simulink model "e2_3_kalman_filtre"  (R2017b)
settings: Solver=FixedStepAuto  StartTime=0.0  StopTime=30  FixedStep=fixed_step_size  RelTol=1e-3
StopFcn:
  | if AUTOLAND
  | %1_2
  | land1 = rospublisher('/tello1/land','std_msgs/Empty');
  | msg=rosmessage(land1);
  | send(land1,msg);
  | land2 = rospublisher('/tello2/land','std_msgs/Empty');
  | msg=rosmessage(land2);
  | send(land2,msg);
  | %3_4
  | land3 = rospublisher('/tello3/land','std_msgs/Empty');
  | msg=rosmessage(land3);
  | send(land3,msg);
  | land4 = rospublisher('/tello4/land','std_msgs/Empty');
  | msg=rosmessage(land4);
  | send(land4,msg);
  | %5_6
  | land5 = rospublisher('/tello5/land','std_msgs/Empty');
  | msg=rosmessage(land5);
  | send(land5,msg);
  | land6= rospublisher('/tello6/land','std_msgs/Empty');
  | msg=rosmessage(land6);
  | send(land6,msg);
  | %7_8
  | land7 = rospublisher('/tello7/land','std_msgs/Empty');
  | msg=rosmessage(land7);
  | send(land7,msg);
  | land8 = rospublisher('/tello8/land','std_msgs/Empty');
  | msg=rosmessage(land8);
  | send(land8,msg);
  | end
  | 
  | generate_cifer_datapack
  | 
  | if TELLO_PLOT
  | tello8_plot
  | end
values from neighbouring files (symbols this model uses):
  a = XMAX    (= 0.8)    [start_tello.m]
  b = YMAX    (= 1.2)    [start_tello.m]
  battery_threshold = 15    [start_tello.m]
  bb = (ZMIN*YMAX - ZMAX*YMIN)/(YMAX - YMIN)    (= -1.05)    [start_tello.m]
  fcnCmdMag = 1    [start.m]
  fcnNumber = 4    [start.m]
  fcnSinFreq = 50.0    (= 50)    [start.m]
  high_time = 5    [start.m]
  k = (ZMAX - ZMIN)/(YMAX - YMIN)    (= 0.458333333333)    [start_tello.m]
  omega = 1.0    (= 1)    [start.m]    (also in start_tello.m = 0.3)
  PARAM_C1 = 4.0    (= 4)    [start.m]
  PARAM_C2 = 0.0187    [start.m]
  PARAM_isNoiseOn = false    [start.m]
  PARAM_T_rec = ceil(5*2*pi/PARAM_w_min)    [start.m]
  PARAM_time_end = PARAM_time_start + 20    (= 23)    [start.m]
  PARAM_time_start = 3    [start.m]
  PARAM_w_max = 12    [start.m]
  PARAM_w_min = 0.5    [start.m]
  R = 1.0    (= 1)    [start.m]    (also in start_tello.m)
  sim_end_time = 15*act_end + 4    (= 475.238898038)    [start_tello.m]
  step_period = zero1_time+high_time+zero2_time+low_time    (= 18)    [start.m]
  tb2 = tb    (= 2.7)    [start_tello.m]
  tb3 = tb*2    (= 5.4)    [start_tello.m]
  tb4 = tb*3    (= 8.1)    [start_tello.m]
  tb5 = tb*4    (= 10.8)    [start_tello.m]
  tb6 = tb*5    (= 13.5)    [start_tello.m]
  tb7 = tb*6    (= 16.2)    [start_tello.m]
  tb8 = tb*7    (= 18.9)    [start_tello.m]
  TELLO1_NUM = uint8(1)    [start_tello.m]
  TELLO2_NUM = uint8(2)    [start_tello.m]
  TELLO3_NUM = uint8(3)    [start_tello.m]
  TELLO4_NUM = uint8(4)    [start_tello.m]
  TELLO5_NUM = uint8(5)    [start_tello.m]
  TELLO6_NUM = uint8(6)    [start_tello.m]
  TELLO7_NUM = uint8(7)    [start_tello.m]
  TELLO8_NUM = uint8(8)    [start_tello.m]
  UAV_NUM = 0    [start_tello.m]
  w1 = 0.4    [start_tello.m]
  w2 = 0.2    [start_tello.m]
  z_d_for_land = -0.2    [start_tello.m]
  zero1_time = 3    [start.m]
  zero2_time = 5    [start.m]
  zero3_time = 5    [start.m]
undefined symbols (not defined in the file or in its folder): DiscIntNeverNeededParam, sigbuilder_block
libraries: simulink x45, etargetslib x24, dspnetwork x24, sharedtransform x8, aerolibanimutils x1
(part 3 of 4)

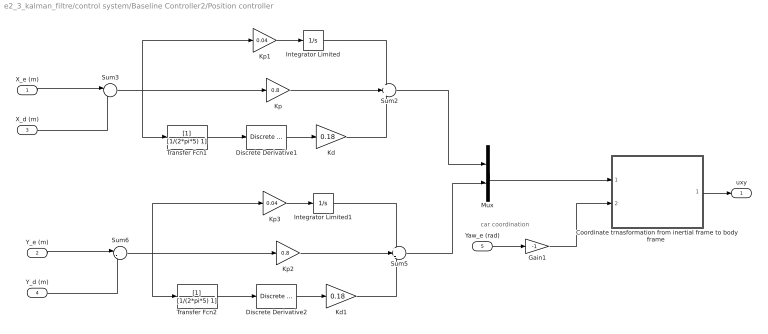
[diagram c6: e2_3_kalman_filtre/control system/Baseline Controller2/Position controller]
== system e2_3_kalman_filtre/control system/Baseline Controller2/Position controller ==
  note: car coordination
  X_e (m) : Inport
  Y_e (m) : Inport  Port=2
  X_d (m) : Inport  Port=3
  Y_d (m) : Inport  Port=4
  Yaw_e (rad) : Inport  Port=5
  "Coordinate trnasformation from inertial frame to body frame " : MATLAB Function  TreatAsAtomicUnit=on
  Discrete Derivative1 : simulink/Discrete/Discrete Derivative  gainval=1.0  ICPrevScaledInput=0.0  OutMin=[]  OutMax=[]  OutDataType=fixdt(1, 16)  OutScaling=2^-10  DoSatur=off
  Discrete Derivative2 : simulink/Discrete/Discrete Derivative  gainval=1.0  ICPrevScaledInput=0.0  OutMin=[]  OutMax=[]  OutDataType=fixdt(1, 16)  OutScaling=2^-10  DoSatur=off
  Gain1 : Gain  Gain=-1
  Integrator Limited : Integrator  LimitOutput=on  UpperSaturationLimit=0.5  LowerSaturationLimit=-0.5
  Integrator Limited1 : Integrator  LimitOutput=on  UpperSaturationLimit=0.5  LowerSaturationLimit=-0.5
  Kd : Gain  Gain=0.18
  Kd1 : Gain  Gain=0.18
  Kp : Gain  Gain=0.8
  Kp1 : Gain  Gain=0.04
  Kp2 : Gain  Gain=0.8
  Kp3 : Gain  Gain=0.04
  Mux : Mux  Inputs=2
  Sum2 : Sum  Inputs=+++
  Sum3 : Sum  Inputs=|-+
  Sum5 : Sum  Inputs=+++
  Sum6 : Sum  Inputs=|-+
  Transfer Fcn1 : TransferFcn  Denominator=[1/(2*pi*5) 1]
  Transfer Fcn2 : TransferFcn  Denominator=[1/(2*pi*5) 1]
  uxy : Outport
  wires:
  Sum6/1 -> Transfer Fcn2/1, Kp3/1, Kp2/1
  Discrete Derivative2/1 -> Kd1/1
  Kd1/1 -> Sum5/3
  Transfer Fcn2/1 -> Discrete Derivative2/1
  Y_d (m)/1 -> Sum6/2
  Transfer Fcn1/1 -> Discrete Derivative1/1
  Kd/1 -> Sum2/3
  Discrete Derivative1/1 -> Kd/1
  Sum3/1 -> Kp1/1, Transfer Fcn1/1, Kp/1
  X_d (m)/1 -> Sum3/2
  "Coordinate trnasformation from inertial frame to body frame "/1(Vec_xy) -> uxy/1
  Gain1/1 -> "Coordinate trnasformation from inertial frame to body frame "/2(psi)
  Mux/1 -> "Coordinate trnasformation from inertial frame to body frame "/1(Vec_i)
  Kp3/1 -> Integrator Limited1/1
  Sum5/1 -> Mux/2
  Integrator Limited1/1 -> Sum5/1
  Y_e (m)/1 -> Sum6/1
  Kp2/1 -> Sum5/2
  Kp/1 -> Sum2/2
  Kp1/1 -> Integrator Limited/1
  Sum2/1 -> Mux/1
  Integrator Limited/1 -> Sum2/1
  X_e (m)/1 -> Sum3/1
  Yaw_e (rad)/1 -> Gain1/1

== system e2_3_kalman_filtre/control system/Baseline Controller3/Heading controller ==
  yaw_e (rad) : Inport
  yaw_d. (rad) : Inport  Port=2
  Integrator Limited : Integrator  Commented=on  LimitOutput=on  UpperSaturationLimit=0.3  LowerSaturationLimit=-0.3
  Ki : Gain  Commented=on  Gain=0.01
  Sum1 : Sum  Inputs=|-+
  Sum2 : Sum  Inputs=|++
  proportional control gain - yaw : Gain  Gain=1.0
  yaw_rate_d. (rad/s) : Outport
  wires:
  Sum1/1 -> Ki/1, proportional control gain - yaw/1
  yaw_e (rad)/1 -> Sum1/1
  yaw_d. (rad)/1 -> Sum1/2
  proportional control gain - yaw/1 -> Sum2/1
  Integrator Limited/1 -> Sum2/2
  Ki/1 -> Integrator Limited/1
  Sum2/1 -> yaw_rate_d. (rad/s)/1

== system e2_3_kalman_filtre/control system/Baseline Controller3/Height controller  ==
  Z_d. (m) : Inport
  Z_e (m) : Inport  Port=2
  V_z : Inport  Port=3
  Integrator Limited : Integrator  LimitOutput=on  UpperSaturationLimit=0.5  LowerSaturationLimit=-0.5
  Kd : Gain  Gain=0.01
  Kp : Gain  Gain=1.0
  Kp1 : Gain  Gain=0.01
  Sum1 : Sum  Inputs=|-+
  Sum2 : Sum  Inputs=+++
  Sum3 : Sum  Inputs=|-+
  Transfer Fcn1 : TransferFcn  Denominator=[1/(2*pi*10) 1]
  Z_velocity_d (m/s) : Outport
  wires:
  Sum3/1 -> Kp1/1, Kp/1
  Z_e (m)/1 -> Sum3/1
  V_z/1 -> Transfer Fcn1/1
  Sum1/1 -> Kd/1
  Sum2/1 -> Z_velocity_d (m/s)/1
  Kp/1 -> Sum2/2
  Kd/1 -> Sum2/3
  Kp1/1 -> Integrator Limited/1
  Integrator Limited/1 -> Sum2/1
  Transfer Fcn1/1 -> Sum1/1
  Z_d. (m)/1 -> Sum3/2

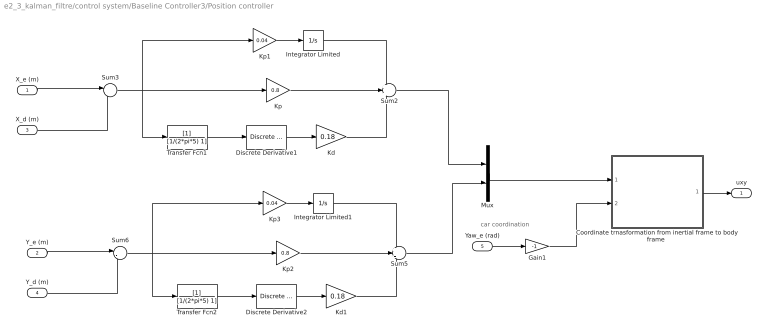
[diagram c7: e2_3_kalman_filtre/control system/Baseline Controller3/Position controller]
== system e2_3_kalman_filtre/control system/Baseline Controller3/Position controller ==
  note: car coordination
  X_e (m) : Inport
  Y_e (m) : Inport  Port=2
  X_d (m) : Inport  Port=3
  Y_d (m) : Inport  Port=4
  Yaw_e (rad) : Inport  Port=5
  "Coordinate trnasformation from inertial frame to body frame " : MATLAB Function  TreatAsAtomicUnit=on
  Discrete Derivative1 : simulink/Discrete/Discrete Derivative  gainval=1.0  ICPrevScaledInput=0.0  OutMin=[]  OutMax=[]  OutDataType=fixdt(1, 16)  OutScaling=2^-10  DoSatur=off
  Discrete Derivative2 : simulink/Discrete/Discrete Derivative  gainval=1.0  ICPrevScaledInput=0.0  OutMin=[]  OutMax=[]  OutDataType=fixdt(1, 16)  OutScaling=2^-10  DoSatur=off
  Gain1 : Gain  Gain=-1
  Integrator Limited : Integrator  LimitOutput=on  UpperSaturationLimit=0.5  LowerSaturationLimit=-0.5
  Integrator Limited1 : Integrator  LimitOutput=on  UpperSaturationLimit=0.5  LowerSaturationLimit=-0.5
  Kd : Gain  Gain=0.18
  Kd1 : Gain  Gain=0.18
  Kp : Gain  Gain=0.8
  Kp1 : Gain  Gain=0.04
  Kp2 : Gain  Gain=0.8
  Kp3 : Gain  Gain=0.04
  Mux : Mux  Inputs=2
  Sum2 : Sum  Inputs=+++
  Sum3 : Sum  Inputs=|-+
  Sum5 : Sum  Inputs=+++
  Sum6 : Sum  Inputs=|-+
  Transfer Fcn1 : TransferFcn  Denominator=[1/(2*pi*5) 1]
  Transfer Fcn2 : TransferFcn  Denominator=[1/(2*pi*5) 1]
  uxy : Outport
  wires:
  Yaw_e (rad)/1 -> Gain1/1
  X_e (m)/1 -> Sum3/1
  Integrator Limited/1 -> Sum2/1
  Sum2/1 -> Mux/1
  Kp1/1 -> Integrator Limited/1
  Kp/1 -> Sum2/2
  Kp2/1 -> Sum5/2
  Y_e (m)/1 -> Sum6/1
  Integrator Limited1/1 -> Sum5/1
  Sum5/1 -> Mux/2
  Kp3/1 -> Integrator Limited1/1
  Mux/1 -> "Coordinate trnasformation from inertial frame to body frame "/1(Vec_i)
  Gain1/1 -> "Coordinate trnasformation from inertial frame to body frame "/2(psi)
  "Coordinate trnasformation from inertial frame to body frame "/1(Vec_xy) -> uxy/1
  X_d (m)/1 -> Sum3/2
  Sum3/1 -> Kp/1, Transfer Fcn1/1, Kp1/1
  Discrete Derivative1/1 -> Kd/1
  Kd/1 -> Sum2/3
  Transfer Fcn1/1 -> Discrete Derivative1/1
  Y_d (m)/1 -> Sum6/2
  Transfer Fcn2/1 -> Discrete Derivative2/1
  Kd1/1 -> Sum5/3
  Discrete Derivative2/1 -> Kd1/1
  Sum6/1 -> Kp2/1, Kp3/1, Transfer Fcn2/1

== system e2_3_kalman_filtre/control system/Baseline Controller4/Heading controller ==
  yaw_e (rad) : Inport
  yaw_d. (rad) : Inport  Port=2
  Integrator Limited : Integrator  Commented=on  LimitOutput=on  UpperSaturationLimit=0.3  LowerSaturationLimit=-0.3
  Ki : Gain  Commented=on  Gain=0.01
  Sum1 : Sum  Inputs=|-+
  Sum2 : Sum  Inputs=|++
  proportional control gain - yaw : Gain  Gain=1.0
  yaw_rate_d. (rad/s) : Outport
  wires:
  Sum2/1 -> yaw_rate_d. (rad/s)/1
  Ki/1 -> Integrator Limited/1
  Integrator Limited/1 -> Sum2/2
  proportional control gain - yaw/1 -> Sum2/1
  yaw_d. (rad)/1 -> Sum1/2
  yaw_e (rad)/1 -> Sum1/1
  Sum1/1 -> proportional control gain - yaw/1, Ki/1

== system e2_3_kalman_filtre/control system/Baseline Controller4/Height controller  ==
  Z_d. (m) : Inport
  Z_e (m) : Inport  Port=2
  V_z : Inport  Port=3
  Integrator Limited : Integrator  LimitOutput=on  UpperSaturationLimit=0.5  LowerSaturationLimit=-0.5
  Kd : Gain  Gain=0.01
  Kp : Gain  Gain=1.0
  Kp1 : Gain  Gain=0.01
  Sum1 : Sum  Inputs=|-+
  Sum2 : Sum  Inputs=+++
  Sum3 : Sum  Inputs=|-+
  Transfer Fcn1 : TransferFcn  Denominator=[1/(2*pi*10) 1]
  Z_velocity_d (m/s) : Outport
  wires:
  Z_d. (m)/1 -> Sum3/2
  Transfer Fcn1/1 -> Sum1/1
  Integrator Limited/1 -> Sum2/1
  Kp1/1 -> Integrator Limited/1
  Kd/1 -> Sum2/3
  Kp/1 -> Sum2/2
  Sum2/1 -> Z_velocity_d (m/s)/1
  Sum1/1 -> Kd/1
  V_z/1 -> Transfer Fcn1/1
  Z_e (m)/1 -> Sum3/1
  Sum3/1 -> Kp/1, Kp1/1

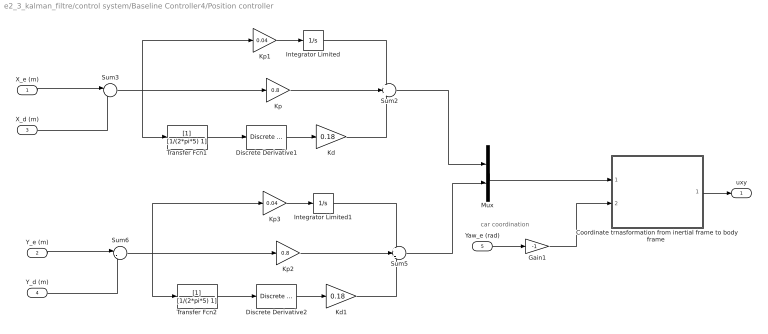
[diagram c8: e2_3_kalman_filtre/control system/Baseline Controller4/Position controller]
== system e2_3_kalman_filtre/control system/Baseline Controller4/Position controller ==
  note: car coordination
  X_e (m) : Inport
  Y_e (m) : Inport  Port=2
  X_d (m) : Inport  Port=3
  Y_d (m) : Inport  Port=4
  Yaw_e (rad) : Inport  Port=5
  "Coordinate trnasformation from inertial frame to body frame " : MATLAB Function  TreatAsAtomicUnit=on
  Discrete Derivative1 : simulink/Discrete/Discrete Derivative  gainval=1.0  ICPrevScaledInput=0.0  OutMin=[]  OutMax=[]  OutDataType=fixdt(1, 16)  OutScaling=2^-10  DoSatur=off
  Discrete Derivative2 : simulink/Discrete/Discrete Derivative  gainval=1.0  ICPrevScaledInput=0.0  OutMin=[]  OutMax=[]  OutDataType=fixdt(1, 16)  OutScaling=2^-10  DoSatur=off
  Gain1 : Gain  Gain=-1
  Integrator Limited : Integrator  LimitOutput=on  UpperSaturationLimit=0.5  LowerSaturationLimit=-0.5
  Integrator Limited1 : Integrator  LimitOutput=on  UpperSaturationLimit=0.5  LowerSaturationLimit=-0.5
  Kd : Gain  Gain=0.18
  Kd1 : Gain  Gain=0.18
  Kp : Gain  Gain=0.8
  Kp1 : Gain  Gain=0.04
  Kp2 : Gain  Gain=0.8
  Kp3 : Gain  Gain=0.04
  Mux : Mux  Inputs=2
  Sum2 : Sum  Inputs=+++
  Sum3 : Sum  Inputs=|-+
  Sum5 : Sum  Inputs=+++
  Sum6 : Sum  Inputs=|-+
  Transfer Fcn1 : TransferFcn  Denominator=[1/(2*pi*5) 1]
  Transfer Fcn2 : TransferFcn  Denominator=[1/(2*pi*5) 1]
  uxy : Outport
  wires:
  Sum6/1 -> Transfer Fcn2/1, Kp3/1, Kp2/1
  Discrete Derivative2/1 -> Kd1/1
  Kd1/1 -> Sum5/3
  Transfer Fcn2/1 -> Discrete Derivative2/1
  Y_d (m)/1 -> Sum6/2
  Transfer Fcn1/1 -> Discrete Derivative1/1
  Kd/1 -> Sum2/3
  Discrete Derivative1/1 -> Kd/1
  Sum3/1 -> Kp1/1, Transfer Fcn1/1, Kp/1
  X_d (m)/1 -> Sum3/2
  "Coordinate trnasformation from inertial frame to body frame "/1(Vec_xy) -> uxy/1
  Gain1/1 -> "Coordinate trnasformation from inertial frame to body frame "/2(psi)
  Mux/1 -> "Coordinate trnasformation from inertial frame to body frame "/1(Vec_i)
  Kp3/1 -> Integrator Limited1/1
  Sum5/1 -> Mux/2
  Integrator Limited1/1 -> Sum5/1
  Y_e (m)/1 -> Sum6/1
  Kp2/1 -> Sum5/2
  Kp/1 -> Sum2/2
  Kp1/1 -> Integrator Limited/1
  Sum2/1 -> Mux/1
  Integrator Limited/1 -> Sum2/1
  X_e (m)/1 -> Sum3/1
  Yaw_e (rad)/1 -> Gain1/1

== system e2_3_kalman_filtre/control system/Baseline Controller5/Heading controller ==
  yaw_e (rad) : Inport
  yaw_d. (rad) : Inport  Port=2
  Integrator Limited : Integrator  Commented=on  LimitOutput=on  UpperSaturationLimit=0.3  LowerSaturationLimit=-0.3
  Ki : Gain  Commented=on  Gain=0.01
  Sum1 : Sum  Inputs=|-+
  Sum2 : Sum  Inputs=|++
  proportional control gain - yaw : Gain  Gain=1.0
  yaw_rate_d. (rad/s) : Outport
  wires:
  Sum1/1 -> Ki/1, proportional control gain - yaw/1
  yaw_e (rad)/1 -> Sum1/1
  yaw_d. (rad)/1 -> Sum1/2
  proportional control gain - yaw/1 -> Sum2/1
  Integrator Limited/1 -> Sum2/2
  Ki/1 -> Integrator Limited/1
  Sum2/1 -> yaw_rate_d. (rad/s)/1

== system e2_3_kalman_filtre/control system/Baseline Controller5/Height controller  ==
  Z_d. (m) : Inport
  Z_e (m) : Inport  Port=2
  V_z : Inport  Port=3
  Integrator Limited : Integrator  LimitOutput=on  UpperSaturationLimit=0.5  LowerSaturationLimit=-0.5
  Kd : Gain  Gain=0.01
  Kp : Gain  Gain=1.0
  Kp1 : Gain  Gain=0.01
  Sum1 : Sum  Inputs=|-+
  Sum2 : Sum  Inputs=+++
  Sum3 : Sum  Inputs=|-+
  Transfer Fcn1 : TransferFcn  Denominator=[1/(2*pi*10) 1]
  Z_velocity_d (m/s) : Outport
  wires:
  Sum3/1 -> Kp1/1, Kp/1
  Z_e (m)/1 -> Sum3/1
  V_z/1 -> Transfer Fcn1/1
  Sum1/1 -> Kd/1
  Sum2/1 -> Z_velocity_d (m/s)/1
  Kp/1 -> Sum2/2
  Kd/1 -> Sum2/3
  Kp1/1 -> Integrator Limited/1
  Integrator Limited/1 -> Sum2/1
  Transfer Fcn1/1 -> Sum1/1
  Z_d. (m)/1 -> Sum3/2

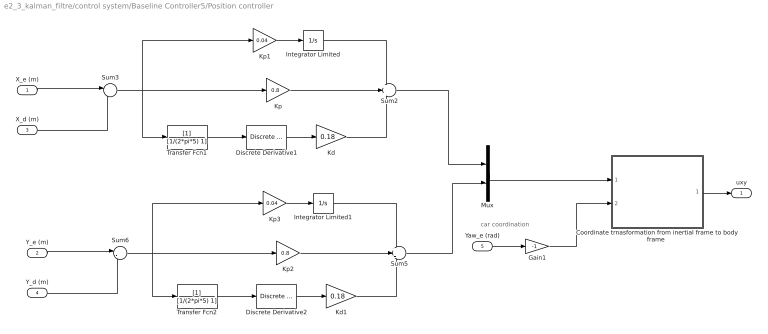
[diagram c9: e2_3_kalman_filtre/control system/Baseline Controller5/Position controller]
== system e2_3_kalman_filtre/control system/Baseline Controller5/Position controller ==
  note: car coordination
  X_e (m) : Inport
  Y_e (m) : Inport  Port=2
  X_d (m) : Inport  Port=3
  Y_d (m) : Inport  Port=4
  Yaw_e (rad) : Inport  Port=5
  "Coordinate trnasformation from inertial frame to body frame " : MATLAB Function  TreatAsAtomicUnit=on
  Discrete Derivative1 : simulink/Discrete/Discrete Derivative  gainval=1.0  ICPrevScaledInput=0.0  OutMin=[]  OutMax=[]  OutDataType=fixdt(1, 16)  OutScaling=2^-10  DoSatur=off
  Discrete Derivative2 : simulink/Discrete/Discrete Derivative  gainval=1.0  ICPrevScaledInput=0.0  OutMin=[]  OutMax=[]  OutDataType=fixdt(1, 16)  OutScaling=2^-10  DoSatur=off
  Gain1 : Gain  Gain=-1
  Integrator Limited : Integrator  LimitOutput=on  UpperSaturationLimit=0.5  LowerSaturationLimit=-0.5
  Integrator Limited1 : Integrator  LimitOutput=on  UpperSaturationLimit=0.5  LowerSaturationLimit=-0.5
  Kd : Gain  Gain=0.18
  Kd1 : Gain  Gain=0.18
  Kp : Gain  Gain=0.8
  Kp1 : Gain  Gain=0.04
  Kp2 : Gain  Gain=0.8
  Kp3 : Gain  Gain=0.04
  Mux : Mux  Inputs=2
  Sum2 : Sum  Inputs=+++
  Sum3 : Sum  Inputs=|-+
  Sum5 : Sum  Inputs=+++
  Sum6 : Sum  Inputs=|-+
  Transfer Fcn1 : TransferFcn  Denominator=[1/(2*pi*5) 1]
  Transfer Fcn2 : TransferFcn  Denominator=[1/(2*pi*5) 1]
  uxy : Outport
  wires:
  Yaw_e (rad)/1 -> Gain1/1
  X_e (m)/1 -> Sum3/1
  Integrator Limited/1 -> Sum2/1
  Sum2/1 -> Mux/1
  Kp1/1 -> Integrator Limited/1
  Kp/1 -> Sum2/2
  Kp2/1 -> Sum5/2
  Y_e (m)/1 -> Sum6/1
  Integrator Limited1/1 -> Sum5/1
  Sum5/1 -> Mux/2
  Kp3/1 -> Integrator Limited1/1
  Mux/1 -> "Coordinate trnasformation from inertial frame to body frame "/1(Vec_i)
  Gain1/1 -> "Coordinate trnasformation from inertial frame to body frame "/2(psi)
  "Coordinate trnasformation from inertial frame to body frame "/1(Vec_xy) -> uxy/1
  X_d (m)/1 -> Sum3/2
  Sum3/1 -> Kp/1, Transfer Fcn1/1, Kp1/1
  Discrete Derivative1/1 -> Kd/1
  Kd/1 -> Sum2/3
  Transfer Fcn1/1 -> Discrete Derivative1/1
  Y_d (m)/1 -> Sum6/2
  Transfer Fcn2/1 -> Discrete Derivative2/1
  Kd1/1 -> Sum5/3
  Discrete Derivative2/1 -> Kd1/1
  Sum6/1 -> Kp2/1, Kp3/1, Transfer Fcn2/1

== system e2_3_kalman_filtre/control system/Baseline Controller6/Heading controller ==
  yaw_e (rad) : Inport
  yaw_d. (rad) : Inport  Port=2
  Integrator Limited : Integrator  Commented=on  LimitOutput=on  UpperSaturationLimit=0.3  LowerSaturationLimit=-0.3
  Ki : Gain  Commented=on  Gain=0.01
  Sum1 : Sum  Inputs=|-+
  Sum2 : Sum  Inputs=|++
  proportional control gain - yaw : Gain  Gain=1.0
  yaw_rate_d. (rad/s) : Outport
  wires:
  Sum2/1 -> yaw_rate_d. (rad/s)/1
  Ki/1 -> Integrator Limited/1
  Integrator Limited/1 -> Sum2/2
  proportional control gain - yaw/1 -> Sum2/1
  yaw_d. (rad)/1 -> Sum1/2
  yaw_e (rad)/1 -> Sum1/1
  Sum1/1 -> proportional control gain - yaw/1, Ki/1

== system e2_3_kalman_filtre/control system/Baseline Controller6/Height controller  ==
  Z_d. (m) : Inport
  Z_e (m) : Inport  Port=2
  V_z : Inport  Port=3
  Integrator Limited : Integrator  LimitOutput=on  UpperSaturationLimit=0.5  LowerSaturationLimit=-0.5
  Kd : Gain  Gain=0.01
  Kp : Gain  Gain=1.0
  Kp1 : Gain  Gain=0.01
  Sum1 : Sum  Inputs=|-+
  Sum2 : Sum  Inputs=+++
  Sum3 : Sum  Inputs=|-+
  Transfer Fcn1 : TransferFcn  Denominator=[1/(2*pi*10) 1]
  Z_velocity_d (m/s) : Outport
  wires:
  Z_d. (m)/1 -> Sum3/2
  Transfer Fcn1/1 -> Sum1/1
  Integrator Limited/1 -> Sum2/1
  Kp1/1 -> Integrator Limited/1
  Kd/1 -> Sum2/3
  Kp/1 -> Sum2/2
  Sum2/1 -> Z_velocity_d (m/s)/1
  Sum1/1 -> Kd/1
  V_z/1 -> Transfer Fcn1/1
  Z_e (m)/1 -> Sum3/1
  Sum3/1 -> Kp/1, Kp1/1

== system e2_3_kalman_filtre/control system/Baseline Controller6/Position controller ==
  note: car coordination
  X_e (m) : Inport
  Y_e (m) : Inport  Port=2
  X_d (m) : Inport  Port=3
  Y_d (m) : Inport  Port=4
  Yaw_e (rad) : Inport  Port=5
  "Coordinate trnasformation from inertial frame to body frame " : MATLAB Function  TreatAsAtomicUnit=on
  Discrete Derivative1 : simulink/Discrete/Discrete Derivative  gainval=1.0  ICPrevScaledInput=0.0  OutMin=[]  OutMax=[]  OutDataType=fixdt(1, 16)  OutScaling=2^-10  DoSatur=off
  Discrete Derivative2 : simulink/Discrete/Discrete Derivative  gainval=1.0  ICPrevScaledInput=0.0  OutMin=[]  OutMax=[]  OutDataType=fixdt(1, 16)  OutScaling=2^-10  DoSatur=off
  Gain1 : Gain  Gain=-1
  Integrator Limited : Integrator  LimitOutput=on  UpperSaturationLimit=0.5  LowerSaturationLimit=-0.5
  Integrator Limited1 : Integrator  LimitOutput=on  UpperSaturationLimit=0.5  LowerSaturationLimit=-0.5
  Kd : Gain  Gain=0.18
  Kd1 : Gain  Gain=0.18
  Kp : Gain  Gain=0.8
  Kp1 : Gain  Gain=0.04
  Kp2 : Gain  Gain=0.8
  Kp3 : Gain  Gain=0.04
  Mux : Mux  Inputs=2
  Sum2 : Sum  Inputs=+++
  Sum3 : Sum  Inputs=|-+
  Sum5 : Sum  Inputs=+++
  Sum6 : Sum  Inputs=|-+
  Transfer Fcn1 : TransferFcn  Denominator=[1/(2*pi*5) 1]
  Transfer Fcn2 : TransferFcn  Denominator=[1/(2*pi*5) 1]
  uxy : Outport
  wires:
  Sum6/1 -> Transfer Fcn2/1, Kp3/1, Kp2/1
  Discrete Derivative2/1 -> Kd1/1
  Kd1/1 -> Sum5/3
  Transfer Fcn2/1 -> Discrete Derivative2/1
  Y_d (m)/1 -> Sum6/2
  Transfer Fcn1/1 -> Discrete Derivative1/1
  Kd/1 -> Sum2/3
  Discrete Derivative1/1 -> Kd/1
  Sum3/1 -> Kp1/1, Transfer Fcn1/1, Kp/1
  X_d (m)/1 -> Sum3/2
  "Coordinate trnasformation from inertial frame to body frame "/1(Vec_xy) -> uxy/1
  Gain1/1 -> "Coordinate trnasformation from inertial frame to body frame "/2(psi)
  Mux/1 -> "Coordinate trnasformation from inertial frame to body frame "/1(Vec_i)
  Kp3/1 -> Integrator Limited1/1
  Sum5/1 -> Mux/2
  Integrator Limited1/1 -> Sum5/1
  Y_e (m)/1 -> Sum6/1
  Kp2/1 -> Sum5/2
  Kp/1 -> Sum2/2
  Kp1/1 -> Integrator Limited/1
  Sum2/1 -> Mux/1
  Integrator Limited/1 -> Sum2/1
  X_e (m)/1 -> Sum3/1
  Yaw_e (rad)/1 -> Gain1/1

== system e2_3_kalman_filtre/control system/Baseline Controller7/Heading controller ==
  yaw_e (rad) : Inport
  yaw_d. (rad) : Inport  Port=2
  Integrator Limited : Integrator  Commented=on  LimitOutput=on  UpperSaturationLimit=0.3  LowerSaturationLimit=-0.3
  Ki : Gain  Commented=on  Gain=0.01
  Sum1 : Sum  Inputs=|-+
  Sum2 : Sum  Inputs=|++
  proportional control gain - yaw : Gain  Gain=1.0
  yaw_rate_d. (rad/s) : Outport
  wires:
  Sum1/1 -> Ki/1, proportional control gain - yaw/1
  yaw_e (rad)/1 -> Sum1/1
  yaw_d. (rad)/1 -> Sum1/2
  proportional control gain - yaw/1 -> Sum2/1
  Integrator Limited/1 -> Sum2/2
  Ki/1 -> Integrator Limited/1
  Sum2/1 -> yaw_rate_d. (rad/s)/1

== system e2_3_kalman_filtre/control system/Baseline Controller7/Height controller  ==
  Z_d. (m) : Inport
  Z_e (m) : Inport  Port=2
  V_z : Inport  Port=3
  Integrator Limited : Integrator  LimitOutput=on  UpperSaturationLimit=0.5  LowerSaturationLimit=-0.5
  Kd : Gain  Gain=0.01
  Kp : Gain  Gain=1.0
  Kp1 : Gain  Gain=0.01
  Sum1 : Sum  Inputs=|-+
  Sum2 : Sum  Inputs=+++
  Sum3 : Sum  Inputs=|-+
  Transfer Fcn1 : TransferFcn  Denominator=[1/(2*pi*10) 1]
  Z_velocity_d (m/s) : Outport
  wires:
  Sum3/1 -> Kp1/1, Kp/1
  Z_e (m)/1 -> Sum3/1
  V_z/1 -> Transfer Fcn1/1
  Sum1/1 -> Kd/1
  Sum2/1 -> Z_velocity_d (m/s)/1
  Kp/1 -> Sum2/2
  Kd/1 -> Sum2/3
  Kp1/1 -> Integrator Limited/1
  Integrator Limited/1 -> Sum2/1
  Transfer Fcn1/1 -> Sum1/1
  Z_d. (m)/1 -> Sum3/2

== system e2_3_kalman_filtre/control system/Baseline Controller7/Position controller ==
  note: car coordination
  X_e (m) : Inport
  Y_e (m) : Inport  Port=2
  X_d (m) : Inport  Port=3
  Y_d (m) : Inport  Port=4
  Yaw_e (rad) : Inport  Port=5
  "Coordinate trnasformation from inertial frame to body frame " : MATLAB Function  TreatAsAtomicUnit=on
  Discrete Derivative1 : simulink/Discrete/Discrete Derivative  gainval=1.0  ICPrevScaledInput=0.0  OutMin=[]  OutMax=[]  OutDataType=fixdt(1, 16)  OutScaling=2^-10  DoSatur=off
  Discrete Derivative2 : simulink/Discrete/Discrete Derivative  gainval=1.0  ICPrevScaledInput=0.0  OutMin=[]  OutMax=[]  OutDataType=fixdt(1, 16)  OutScaling=2^-10  DoSatur=off
  Gain1 : Gain  Gain=-1
  Integrator Limited : Integrator  LimitOutput=on  UpperSaturationLimit=0.5  LowerSaturationLimit=-0.5
  Integrator Limited1 : Integrator  LimitOutput=on  UpperSaturationLimit=0.5  LowerSaturationLimit=-0.5
  Kd : Gain  Gain=0.18
  Kd1 : Gain  Gain=0.18
  Kp : Gain  Gain=0.8
  Kp1 : Gain  Gain=0.04
  Kp2 : Gain  Gain=0.8
  Kp3 : Gain  Gain=0.04
  Mux : Mux  Inputs=2
  Sum2 : Sum  Inputs=+++
  Sum3 : Sum  Inputs=|-+
  Sum5 : Sum  Inputs=+++
  Sum6 : Sum  Inputs=|-+
  Transfer Fcn1 : TransferFcn  Denominator=[1/(2*pi*5) 1]
  Transfer Fcn2 : TransferFcn  Denominator=[1/(2*pi*5) 1]
  uxy : Outport
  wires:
  Yaw_e (rad)/1 -> Gain1/1
  X_e (m)/1 -> Sum3/1
  Integrator Limited/1 -> Sum2/1
  Sum2/1 -> Mux/1
  Kp1/1 -> Integrator Limited/1
  Kp/1 -> Sum2/2
  Kp2/1 -> Sum5/2
  Y_e (m)/1 -> Sum6/1
  Integrator Limited1/1 -> Sum5/1
  Sum5/1 -> Mux/2
  Kp3/1 -> Integrator Limited1/1
  Mux/1 -> "Coordinate trnasformation from inertial frame to body frame "/1(Vec_i)
  Gain1/1 -> "Coordinate trnasformation from inertial frame to body frame "/2(psi)
  "Coordinate trnasformation from inertial frame to body frame "/1(Vec_xy) -> uxy/1
  X_d (m)/1 -> Sum3/2
  Sum3/1 -> Kp/1, Transfer Fcn1/1, Kp1/1
  Discrete Derivative1/1 -> Kd/1
  Kd/1 -> Sum2/3
  Transfer Fcn1/1 -> Discrete Derivative1/1
  Y_d (m)/1 -> Sum6/2
  Transfer Fcn2/1 -> Discrete Derivative2/1
  Kd1/1 -> Sum5/3
  Discrete Derivative2/1 -> Kd1/1
  Sum6/1 -> Kp2/1, Kp3/1, Transfer Fcn2/1

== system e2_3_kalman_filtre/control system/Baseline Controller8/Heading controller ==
  yaw_e (rad) : Inport
  yaw_d. (rad) : Inport  Port=2
  Integrator Limited : Integrator  Commented=on  LimitOutput=on  UpperSaturationLimit=0.3  LowerSaturationLimit=-0.3
  Ki : Gain  Commented=on  Gain=0.01
  Sum1 : Sum  Inputs=|-+
  Sum2 : Sum  Inputs=|++
  proportional control gain - yaw : Gain  Gain=1.0
  yaw_rate_d. (rad/s) : Outport
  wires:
  Sum2/1 -> yaw_rate_d. (rad/s)/1
  Ki/1 -> Integrator Limited/1
  Integrator Limited/1 -> Sum2/2
  proportional control gain - yaw/1 -> Sum2/1
  yaw_d. (rad)/1 -> Sum1/2
  yaw_e (rad)/1 -> Sum1/1
  Sum1/1 -> proportional control gain - yaw/1, Ki/1

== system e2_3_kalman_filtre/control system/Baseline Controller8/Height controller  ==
  Z_d. (m) : Inport
  Z_e (m) : Inport  Port=2
  V_z : Inport  Port=3
  Integrator Limited : Integrator  LimitOutput=on  UpperSaturationLimit=0.5  LowerSaturationLimit=-0.5
  Kd : Gain  Gain=0.01
  Kp : Gain  Gain=1.0
  Kp1 : Gain  Gain=0.01
  Sum1 : Sum  Inputs=|-+
  Sum2 : Sum  Inputs=+++
  Sum3 : Sum  Inputs=|-+
  Transfer Fcn1 : TransferFcn  Denominator=[1/(2*pi*10) 1]
  Z_velocity_d (m/s) : Outport
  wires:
  Z_d. (m)/1 -> Sum3/2
  Transfer Fcn1/1 -> Sum1/1
  Integrator Limited/1 -> Sum2/1
  Kp1/1 -> Integrator Limited/1
  Kd/1 -> Sum2/3
  Kp/1 -> Sum2/2
  Sum2/1 -> Z_velocity_d (m/s)/1
  Sum1/1 -> Kd/1
  V_z/1 -> Transfer Fcn1/1
  Z_e (m)/1 -> Sum3/1
  Sum3/1 -> Kp/1, Kp1/1

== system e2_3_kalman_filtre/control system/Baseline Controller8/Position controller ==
  note: car coordination
  X_e (m) : Inport
  Y_e (m) : Inport  Port=2
  X_d (m) : Inport  Port=3
  Y_d (m) : Inport  Port=4
  Yaw_e (rad) : Inport  Port=5
  "Coordinate trnasformation from inertial frame to body frame " : MATLAB Function  TreatAsAtomicUnit=on
  Discrete Derivative1 : simulink/Discrete/Discrete Derivative  gainval=1.0  ICPrevScaledInput=0.0  OutMin=[]  OutMax=[]  OutDataType=fixdt(1, 16)  OutScaling=2^-10  DoSatur=off
  Discrete Derivative2 : simulink/Discrete/Discrete Derivative  gainval=1.0  ICPrevScaledInput=0.0  OutMin=[]  OutMax=[]  OutDataType=fixdt(1, 16)  OutScaling=2^-10  DoSatur=off
  Gain1 : Gain  Gain=-1
  Integrator Limited : Integrator  LimitOutput=on  UpperSaturationLimit=0.5  LowerSaturationLimit=-0.5
  Integrator Limited1 : Integrator  LimitOutput=on  UpperSaturationLimit=0.5  LowerSaturationLimit=-0.5
  Kd : Gain  Gain=0.18
  Kd1 : Gain  Gain=0.18
  Kp : Gain  Gain=0.8
  Kp1 : Gain  Gain=0.04
  Kp2 : Gain  Gain=0.8
  Kp3 : Gain  Gain=0.04
  Mux : Mux  Inputs=2
  Sum2 : Sum  Inputs=+++
  Sum3 : Sum  Inputs=|-+
  Sum5 : Sum  Inputs=+++
  Sum6 : Sum  Inputs=|-+
  Transfer Fcn1 : TransferFcn  Denominator=[1/(2*pi*5) 1]
  Transfer Fcn2 : TransferFcn  Denominator=[1/(2*pi*5) 1]
  uxy : Outport
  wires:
  Sum6/1 -> Transfer Fcn2/1, Kp3/1, Kp2/1
  Discrete Derivative2/1 -> Kd1/1
  Kd1/1 -> Sum5/3
  Transfer Fcn2/1 -> Discrete Derivative2/1
  Y_d (m)/1 -> Sum6/2
  Transfer Fcn1/1 -> Discrete Derivative1/1
  Kd/1 -> Sum2/3
  Discrete Derivative1/1 -> Kd/1
  Sum3/1 -> Kp1/1, Transfer Fcn1/1, Kp/1
  X_d (m)/1 -> Sum3/2
  "Coordinate trnasformation from inertial frame to body frame "/1(Vec_xy) -> uxy/1
  Gain1/1 -> "Coordinate trnasformation from inertial frame to body frame "/2(psi)
  Mux/1 -> "Coordinate trnasformation from inertial frame to body frame "/1(Vec_i)
  Kp3/1 -> Integrator Limited1/1
  Sum5/1 -> Mux/2
  Integrator Limited1/1 -> Sum5/1
  Y_e (m)/1 -> Sum6/1
  Kp2/1 -> Sum5/2
  Kp/1 -> Sum2/2
  Kp1/1 -> Integrator Limited/1
  Sum2/1 -> Mux/1
  Integrator Limited/1 -> Sum2/1
  X_e (m)/1 -> Sum3/1
  Yaw_e (rad)/1 -> Gain1/1

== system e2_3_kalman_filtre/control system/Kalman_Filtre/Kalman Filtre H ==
  The system output: Position : Inport
  real_vz : Inport  Port=2
  Demux : Demux  Outputs=9
  Error : Scope
  Kalman Filtre H : Subsystem
  Kalman Filtre for getting the velocity H : MATLAB Function  TreatAsAtomicUnit=on
  Manual Switch1 : ManualSwitch  CurrentSetting=0
  Memory block for resolving the 'algebraic loop' problem : Memory
  Scope2 : Scope
  Scope4 : Scope  NumInputPorts=8
  Sum : Sum  Inputs=-+|
  The comparison of velocity signal between 'Derivative' and 'Kalman filtering' : Scope  NumInputPorts=2
  Unit Delay1 : UnitDelay  SampleTime=-1
  Unit Delay7 : UnitDelay  SampleTime=-1
  Unit Delay8 : UnitDelay  SampleTime=-1
  Zero-Order Hold1 : ZeroOrderHold  SampleTime=-1
  Out velocity feedback : Outport
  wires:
  Kalman Filtre for getting the velocity H/1(Covariance_matrice) -> Scope2/1
  Kalman Filtre for getting the velocity H/2(X_Kalmanfiltred) -> Memory block for resolving the 'algebraic loop' problem/1
  Memory block for resolving the 'algebraic loop' problem/1 -> Demux/1
  Zero-Order Hold1/1 -> Kalman Filtre for getting the velocity H/1(Mesurement_Velocity)
  Manual Switch1/1 -> Out velocity feedback/1
  Demux/1 -> Scope4/1
  The system output: Position/1 -> Kalman Filtre H/1(The system output: Position), Unit Delay7/1
  Demux/2 -> Scope4/2
  Demux/3 -> Scope4/3
  Demux/4 -> Scope4/4
  Demux/5 -> Scope4/5
  Unit Delay8/1 -> Zero-Order Hold1/1
  Demux/6 -> Scope4/6
  Demux/7 -> Scope4/8
  Demux/8 -> Manual Switch1/1, Sum/1, The comparison of velocity signal between 'Derivative' and 'Kalman filtering'/1
  Demux/9 -> Scope4/7
  real_vz/1 -> Manual Switch1/2, The comparison of velocity signal between 'Derivative' and 'Kalman filtering'/2
  Unit Delay7/1 -> Unit Delay1/1
  Unit Delay1/1 -> Unit Delay8/1
  Sum/1 -> Error/1
  Kalman Filtre H/1(Out velocity feedback) -> Sum/2

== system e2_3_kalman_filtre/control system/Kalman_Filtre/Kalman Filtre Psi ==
  The system output: Position : Inport
  real_vpsi : Inport  Port=2
  Demux : Demux  Outputs=9
  Error : Scope
  Kalman Filtre Psi : Subsystem
  Kalman Filtre for getting the velocity Psi : MATLAB Function  TreatAsAtomicUnit=on
  Manual Switch1 : ManualSwitch  CurrentSetting=0
  Memory block for resolving the 'algebraic loop' problem : Memory
  Scope2 : Scope
  Scope4 : Scope  NumInputPorts=8
  Sum : Sum  Inputs=-+|
  The comparison of velocity signal between 'Derivative' and 'Kalman filtering' : Scope  NumInputPorts=2
  Unit Delay1 : UnitDelay  SampleTime=-1
  Unit Delay7 : UnitDelay  SampleTime=-1
  Unit Delay8 : UnitDelay  SampleTime=-1
  Zero-Order Hold1 : ZeroOrderHold  SampleTime=-1
  Out velocity feedback : Outport
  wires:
  Kalman Filtre for getting the velocity Psi/1(Covariance_matrice) -> Scope2/1
  Kalman Filtre for getting the velocity Psi/2(X_Kalmanfiltred) -> Memory block for resolving the 'algebraic loop' problem/1
  Memory block for resolving the 'algebraic loop' problem/1 -> Demux/1
  Zero-Order Hold1/1 -> Kalman Filtre for getting the velocity Psi/1(Mesurement_Velocity)
  Manual Switch1/1 -> Out velocity feedback/1
  Demux/1 -> Scope4/1
  The system output: Position/1 -> Kalman Filtre Psi/1(The system output: Position), Unit Delay7/1
  Demux/2 -> Scope4/2
  Demux/3 -> Scope4/3
  Demux/4 -> Scope4/4
  Demux/5 -> Scope4/5
  Unit Delay8/1 -> Zero-Order Hold1/1
  Demux/6 -> Scope4/6
  Demux/7 -> Scope4/8
  Demux/8 -> Manual Switch1/1, Sum/1, The comparison of velocity signal between 'Derivative' and 'Kalman filtering'/1
  Demux/9 -> Scope4/7
  real_vpsi/1 -> Manual Switch1/2, The comparison of velocity signal between 'Derivative' and 'Kalman filtering'/2
  Unit Delay7/1 -> Unit Delay1/1
  Unit Delay1/1 -> Unit Delay8/1
  Sum/1 -> Error/1
  Kalman Filtre Psi/1(Out velocity feedback) -> Sum/2

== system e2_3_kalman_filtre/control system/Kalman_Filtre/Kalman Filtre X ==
  The system output: Position : Inport
  real_vx : Inport  Port=2
  Demux : Demux  Outputs=9
  Error : Scope
  Kalman Filtre X : Subsystem
  Kalman Filtre for getting the velocity X : MATLAB Function  TreatAsAtomicUnit=on
  Manual Switch1 : ManualSwitch  CurrentSetting=0
  Memory block for resolving the 'algebraic loop' problem : Memory
  Scope : Scope
  Scope4 : Scope  NumInputPorts=8
  Sum : Sum  Inputs=-+|
  The comparison of velocity signal between 'Derivative' and 'Kalman filtering' : Scope  NumInputPorts=3
  Unit Delay{1..2,7..8} (4 alike) : UnitDelay  SampleTime=-1
  Zero-Order Hold1 : ZeroOrderHold  SampleTime=-1
  Out velocity feedback : Outport
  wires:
  Kalman Filtre for getting the velocity X/1(Covariance_matrice) -> Scope/1
  Kalman Filtre for getting the velocity X/2(X_Kalmanfiltred) -> Memory block for resolving the 'algebraic loop' problem/1
  Memory block for resolving the 'algebraic loop' problem/1 -> Demux/1
  Zero-Order Hold1/1 -> Kalman Filtre for getting the velocity X/1(Mesurement_Velocity)
  Manual Switch1/1 -> Out velocity feedback/1
  Demux/1 -> Scope4/1
  The system output: Position/1 -> Kalman Filtre X/1(The system output: Position), Unit Delay7/1
  Demux/2 -> Scope4/2
  Demux/3 -> Scope4/3
  Demux/4 -> Scope4/4
  Demux/5 -> Scope4/5
  Unit Delay7/1 -> Unit Delay8/1
  Unit Delay8/1 -> Unit Delay1/1
  Demux/6 -> Scope4/6
  Demux/7 -> Scope4/8
  Demux/8 -> Manual Switch1/1, Sum/1, The comparison of velocity signal between 'Derivative' and 'Kalman filtering'/1
  Demux/9 -> Scope4/7
  real_vx/1 -> Manual Switch1/2, The comparison of velocity signal between 'Derivative' and 'Kalman filtering'/2
  Unit Delay1/1 -> Unit Delay2/1
  Unit Delay2/1 -> Zero-Order Hold1/1
  Kalman Filtre X/1(Out velocity feedback) -> The comparison of velocity signal between 'Derivative' and 'Kalman filtering'/3, Sum/2
  Sum/1 -> Error/1

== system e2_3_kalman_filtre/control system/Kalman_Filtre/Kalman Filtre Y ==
  The system output: Position : Inport
  real_vy : Inport  Port=2
  Demux : Demux  Outputs=9
  Error : Scope
  Kalman Filtre Y : Subsystem
  Kalman Filtre for getting the velocity Y : MATLAB Function  TreatAsAtomicUnit=on
  Manual Switch1 : ManualSwitch  CurrentSetting=0
  Memory block for resolving the 'algebraic loop' problem : Memory
  Scope2 : Scope
  Scope4 : Scope  NumInputPorts=8
  Sum : Sum  Inputs=-+|
  The comparison of velocity signal between 'Derivative' and 'Kalman filtering' : Scope  NumInputPorts=3
  Unit Delay{1..2,7..8} (4 alike) : UnitDelay  SampleTime=-1
  Zero-Order Hold1 : ZeroOrderHold  SampleTime=-1
  Out velocity feedback : Outport
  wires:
  Kalman Filtre for getting the velocity Y/1(Covariance_matrice) -> Scope2/1
  Kalman Filtre for getting the velocity Y/2(X_Kalmanfiltred) -> Memory block for resolving the 'algebraic loop' problem/1
  Memory block for resolving the 'algebraic loop' problem/1 -> Demux/1
  Zero-Order Hold1/1 -> Kalman Filtre for getting the velocity Y/1(Mesurement_Velocity)
  Manual Switch1/1 -> Out velocity feedback/1
  Demux/1 -> Scope4/1
  The system output: Position/1 -> Kalman Filtre Y/1(The system output: Position), Unit Delay7/1
  Demux/2 -> Scope4/2
  Demux/3 -> Scope4/3
  Demux/4 -> Scope4/4
  Demux/5 -> Scope4/5
  Unit Delay2/1 -> Zero-Order Hold1/1
  Demux/6 -> Scope4/6
  Demux/7 -> Scope4/8
  Demux/8 -> Manual Switch1/1, Sum/1, The comparison of velocity signal between 'Derivative' and 'Kalman filtering'/1
  Demux/9 -> Scope4/7
  real_vy/1 -> Manual Switch1/2, The comparison of velocity signal between 'Derivative' and 'Kalman filtering'/2
  Unit Delay1/1 -> Unit Delay2/1
  Unit Delay8/1 -> Unit Delay1/1
  Unit Delay7/1 -> Unit Delay8/1
  Sum/1 -> Error/1
  Kalman Filtre Y/1(Out velocity feedback) -> The comparison of velocity signal between 'Derivative' and 'Kalman filtering'/3, Sum/2

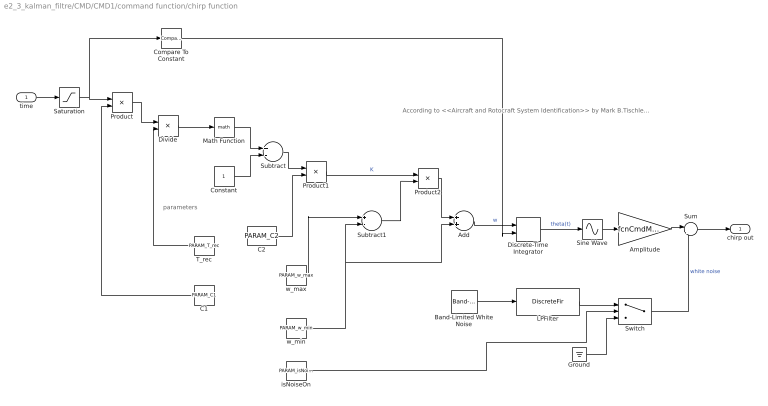
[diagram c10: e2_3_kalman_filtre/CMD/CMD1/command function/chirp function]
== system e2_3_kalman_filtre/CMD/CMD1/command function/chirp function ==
  note: According to <<Aircraft and Rotocraft System Identification>> by Mark B.Tischler, the auto-sweep signal has the following form: signal = A*sin(theta(t) theta(t) = integral(0 to T_rec)(w(t))dt w = w_min + K(w_max - w_min) K = C2*[ exp(C1*t/T_rec) - 1] where C1,C2 is recommened to be 4.0, 0.0187 respectively. Reference values for w_min, w_max, T_rec are 0.3, 12.0, 90. The mentioned formulas can be found in P91, Chapter 5.
  note: parameters
  time : Inport
  Add : Sum
  Amplitude : Gain  Gain=fcnCmdMag
  Band-Limited White Noise : simulink/Sources/Band-Limited White Noise  Cov=1  Ts=0.5  seed=[27891]
  C1 : Constant  Value=PARAM_C1
  C2 : Constant  Value=PARAM_C2
  Compare To Constant : simulink/Logic and Bit Operations/Compare To Constant  relop=<=  const=0  OutDataTypeStr=boolean
  Constant : Constant
  Discrete-Time Integrator : DiscreteIntegrator  gainval=1  ExternalReset=falling  InitialConditionSetting=State (most efficient)  SampleTime=-1  ICPrevOutput=DiscIntNeverNeededParam  ICPrevScaledInput=DiscIntNeverNeededParam
  Divide : Product  Inputs=*/
  Ground : Ground
  LPFilter : DiscreteFir  Tag=BlockMethodSubSystem  Coefficients=[-0.055278305352262344 -0.0018784080618625076 -0.0018600723789761655 -0.0018059014547689388 -0.0017146920181071476 -0.0015871733154672245 -0.0014196557002817895 -0.0012169581089781429 -0.00097448223820069694 -0.0006970439084934615 -0.00037734754437382872 -1.3279419242581616e-05 0.00037595724779108442 0.00081295906181109447 0.0012808192950690851 0.0017881060326839426 0.0023275368728296014 0.0029013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  InputProcessing=Columns as channels (frame based)
  Math Function : Math
  Product : Product
  Product1 : Product
  Product2 : Product
  Saturation : Saturate  UpperLimit=inf  LowerLimit=0
  Sine Wave : Sin  TimeSource=Use external signal  SampleTime=0
  Subtract : Sum  Inputs=+-
  Subtract1 : Sum  Inputs=+-
  Sum : Sum  Inputs=|++
  Switch : Switch  Criteria=u2 > Threshold
  T_rec : Constant  Value=PARAM_T_rec
  isNoiseOn : Constant  Value=PARAM_isNoiseOn
  w_max : Constant  Value=PARAM_w_max
  w_min : Constant  Value=PARAM_w_min
  chirp out : Outport
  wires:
  Compare To Constant/1 -> Discrete-Time Integrator/2
  Saturation/1 -> Product/1, Compare To Constant/1
  isNoiseOn/1 -> Switch/2
  time/1 -> Saturation/1
  LPFilter/1 -> Switch/1
  Switch/1 -> Sum/2  "white noise"
  Ground/1 -> Switch/3
  Band-Limited White Noise/1 -> LPFilter/1
  Sum/1 -> chirp out/1
  Amplitude/1 -> Sum/1
  Discrete-Time Integrator/1 -> Sine Wave/1  "theta(t)"
  Add/1 -> Discrete-Time Integrator/1  "w"
  Sine Wave/1 -> Amplitude/1
  Product2/1 -> Add/1
  Subtract1/1 -> Product2/2
  Product1/1 -> Product2/1  "K"
  w_min/1 -> Subtract1/2, Add/2
  Divide/1 -> Math Function/1
  Subtract/1 -> Product1/1
  Constant/1 -> Subtract/2
  w_max/1 -> Subtract1/1
  C2/1 -> Product1/2
  Math Function/1 -> Subtract/1
  T_rec/1 -> Divide/2
  C1/1 -> Product/2
  Product/1 -> Divide/1

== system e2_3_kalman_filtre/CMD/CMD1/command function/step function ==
  time : Inport
  Constant : Constant  Value=PARAM_time_start
  Constant1 : Constant  Value=PARAM_time_end
  Constant3 : Constant  Value=fcnCmdMag
  Constant4 : Constant  Value=0
  Divide : Product  Inputs=*/
  Divide1 : Product  Inputs=*/
  Gain : Gain  Gain=1/4
  Gain1 : Gain  Gain=3/4
  Subtract : Sum  Inputs=+-
  Switch : Switch  Threshold=1
  Switch1 : Switch  Threshold=1
  stepOut : Outport
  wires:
  Divide1/1 -> Switch1/2
  Divide/1 -> Switch/2
  time/1 -> Divide/1, Divide1/1
  Gain1/1 -> Divide1/2
  Gain/1 -> Divide/2
  Subtract/1 -> Gain1/1, Gain/1  "cmd duration"
  Constant/1 -> Subtract/2
  Constant1/1 -> Subtract/1
  Switch/1 -> Switch1/3
  Switch1/1 -> stepOut/1
  Constant3/1 -> Switch/1
  Constant4/1 -> Switch/3, Switch1/1

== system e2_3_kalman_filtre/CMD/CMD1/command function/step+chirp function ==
  time : Inport
  Switch : Switch  Criteria=u2 > Threshold
  chirp function1 : Subsystem
  step function1 : Subsystem
  Cmd Out : Outport
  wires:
  time/1 -> step function1/1(time)
  step function1/1(timeOut) -> chirp function1/1(time), Switch/2
  Switch/1 -> Cmd Out/1
  step function1/2(stepOut) -> Switch/3
  chirp function1/1(chirp out) -> Switch/1

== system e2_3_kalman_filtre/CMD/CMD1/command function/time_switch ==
  note: param
  input : Inport
  time : Inport  Port=2
  Abs : Abs
  Constant : Constant  Value=0  OutDataTypeStr=single
  Constant3 : Constant  Value=0  OutDataTypeStr=single
  Divide : Product  Inputs=*/
  Divide1 : Product  Inputs=*/
  Switch : Switch  Criteria=u2 > Threshold  Threshold=1
  Switch1 : Switch  Criteria=u2 > Threshold  Threshold=1  OutDataTypeStr=single
  time_end : Constant  Value=PARAM_time_end
  time_start : Constant  Value=PARAM_time_start
  Output : Outport
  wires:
  Divide/1 -> Switch/2
  Divide1/1 -> Switch1/2
  Switch1/1 -> Output/1
  Abs/1 -> Divide1/1, Divide/1
  time/1 -> Abs/1
  time_end/1 -> Divide1/2
  time_start/1 -> Divide/2
  Constant3/1 -> Switch1/1
  Switch/1 -> Switch1/3
  input/1 -> Switch/1
  Constant/1 -> Switch/3

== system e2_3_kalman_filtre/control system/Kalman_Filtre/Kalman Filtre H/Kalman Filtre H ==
  The system output: Position : Inport
  Demux : Demux  Outputs=3
  Kalman Filtre for getting the velocity H : MATLAB Function  TreatAsAtomicUnit=on
  Memory block for resolving the 'algebraic loop' problem : Memory
  Scope2 : Scope
  Scope4 : Scope  NumInputPorts=2
  Out velocity feedback : Outport
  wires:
  Demux/2 -> Out velocity feedback/1
  Memory block for resolving the 'algebraic loop' problem/1 -> Demux/1
  Kalman Filtre for getting the velocity H/1(Covariance_matrice) -> Scope2/1
  The system output: Position/1 -> Kalman Filtre for getting the velocity H/1(Mesurement_Velocity)
  Demux/1 -> Scope4/1
  Kalman Filtre for getting the velocity H/2(X_Kalmanfiltred) -> Memory block for resolving the 'algebraic loop' problem/1
  Demux/3 -> Scope4/2

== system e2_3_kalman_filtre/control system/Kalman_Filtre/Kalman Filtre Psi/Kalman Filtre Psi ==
  The system output: Position : Inport
  Demux : Demux  Outputs=3
  Kalman Filtre for getting the velocity Psi : MATLAB Function  TreatAsAtomicUnit=on
  Memory block for resolving the 'algebraic loop' problem : Memory
  Scope1 : Scope  NumInputPorts=2
  Scope2 : Scope
  Out velocity feedback : Outport
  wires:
  Demux/2 -> Out velocity feedback/1
  Kalman Filtre for getting the velocity Psi/1(Covariance_matrice) -> Scope2/1
  The system output: Position/1 -> Kalman Filtre for getting the velocity Psi/1(Mesurement_Velocity)
  Demux/1 -> Scope1/1
  Demux/3 -> Scope1/2
  Kalman Filtre for getting the velocity Psi/2(X_Kalmanfiltred) -> Memory block for resolving the 'algebraic loop' problem/1
  Memory block for resolving the 'algebraic loop' problem/1 -> Demux/1

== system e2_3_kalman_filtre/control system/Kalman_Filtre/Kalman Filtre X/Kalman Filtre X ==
  The system output: Position : Inport
  Demux : Demux  Outputs=3
  Kalman Filtre for getting the velocity X : MATLAB Function  TreatAsAtomicUnit=on
  Memory block for resolving the 'algebraic loop' problem : Memory
  Scope2 : Scope
  Scope4 : Scope  NumInputPorts=2
  Out velocity feedback : Outport
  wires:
  Kalman Filtre for getting the velocity X/1(Covariance_matrice) -> Scope2/1
  Kalman Filtre for getting the velocity X/2(X_Kalmanfiltred) -> Memory block for resolving the 'algebraic loop' problem/1
  Memory block for resolving the 'algebraic loop' problem/1 -> Demux/1
  The system output: Position/1 -> Kalman Filtre for getting the velocity X/1(Mesurement_Velocity)
  Demux/2 -> Out velocity feedback/1
  Demux/1 -> Scope4/2
  Demux/3 -> Scope4/1

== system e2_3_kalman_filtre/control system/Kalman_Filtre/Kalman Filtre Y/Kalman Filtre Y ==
  The system output: Position : Inport
  Demux : Demux  Outputs=3
  Kalman Filtre for getting the velocity Y : MATLAB Function  TreatAsAtomicUnit=on
  Memory block for resolving the 'algebraic loop' problem : Memory
  Scope2 : Scope
  Scope4 : Scope  NumInputPorts=2
  Out velocity feedback : Outport
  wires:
  Kalman Filtre for getting the velocity Y/2(X_Kalmanfiltred) -> Memory block for resolving the 'algebraic loop' problem/1
  Demux/2 -> Out velocity feedback/1
  Kalman Filtre for getting the velocity Y/1(Covariance_matrice) -> Scope2/1
  Memory block for resolving the 'algebraic loop' problem/1 -> Demux/1
  The system output: Position/1 -> Kalman Filtre for getting the velocity Y/1(Mesurement_Velocity)
  Demux/1 -> Scope4/1
  Demux/3 -> Scope4/2

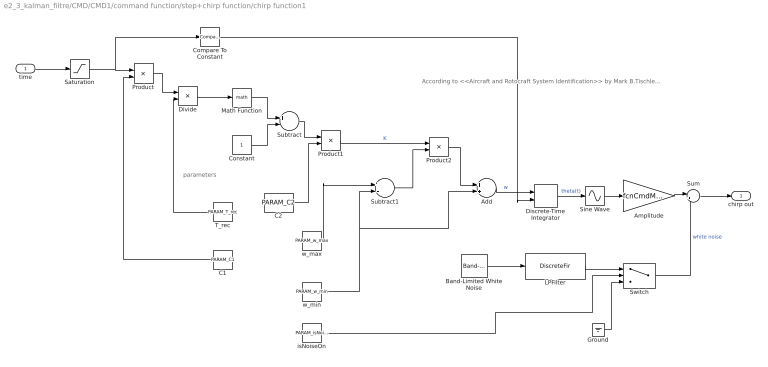
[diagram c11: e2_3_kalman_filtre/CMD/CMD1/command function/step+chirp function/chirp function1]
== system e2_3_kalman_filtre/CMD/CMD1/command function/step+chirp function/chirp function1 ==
  note: parameters
  note: According to <<Aircraft and Rotocraft System Identification>> by Mark B.Tischler, the auto-sweep signal has the following form: signal = A*sin(theta(t) theta(t) = integral(0 to T_rec)(w(t))dt w = w_min + K(w_max - w_min) K = C2*[ exp(C1*t/T_rec) - 1] where C1,C2 is recommened to be 4.0, 0.0187 respectively. Reference values for w_min, w_max, T_rec are 0.3, 12.0, 90. The mentioned formulas can be found in P91, Chapter 5.
  time : Inport
  Add : Sum
  Amplitude : Gain  Gain=fcnCmdMag
  Band-Limited White Noise : simulink/Sources/Band-Limited White Noise  Cov=1  Ts=0.5  seed=[27891]
  C1 : Constant  Value=PARAM_C1
  C2 : Constant  Value=PARAM_C2
  Compare To Constant : simulink/Logic and Bit Operations/Compare To Constant  relop=<=  const=0  OutDataTypeStr=boolean
  Constant : Constant
  Discrete-Time Integrator : DiscreteIntegrator  gainval=1  ExternalReset=falling  InitialConditionSetting=State (most efficient)  SampleTime=-1  ICPrevOutput=DiscIntNeverNeededParam  ICPrevScaledInput=DiscIntNeverNeededParam
  Divide : Product  Inputs=*/
  Ground : Ground
  LPFilter : DiscreteFir  Tag=BlockMethodSubSystem  Coefficients=[-0.055278305352262344 -0.0018784080618625076 -0.0018600723789761655 -0.0018059014547689388 -0.0017146920181071476 -0.0015871733154672245 -0.0014196557002817895 -0.0012169581089781429 -0.00097448223820069694 -0.0006970439084934615 -0.00037734754437382872 -1.3279419242581616e-05 0.00037595724779108442 0.00081295906181109447 0.0012808192950690851 0.0017881060326839426 0.0023275368728296014 0.0029013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  InputProcessing=Columns as channels (frame based)
  Math Function : Math
  Product : Product
  Product1 : Product
  Product2 : Product
  Saturation : Saturate  UpperLimit=inf  LowerLimit=0
  Sine Wave : Sin  TimeSource=Use external signal  SampleTime=0
  Subtract : Sum  Inputs=+-
  Subtract1 : Sum  Inputs=+-
  Sum : Sum  Inputs=|++
  Switch : Switch  Criteria=u2 > Threshold
  T_rec : Constant  Value=PARAM_T_rec
  isNoiseOn : Constant  Value=PARAM_isNoiseOn
  w_max : Constant  Value=PARAM_w_max
  w_min : Constant  Value=PARAM_w_min
  chirp out : Outport
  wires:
  Compare To Constant/1 -> Discrete-Time Integrator/2
  Saturation/1 -> Product/1, Compare To Constant/1
  Product/1 -> Divide/1
  C1/1 -> Product/2
  T_rec/1 -> Divide/2
  Math Function/1 -> Subtract/1
  C2/1 -> Product1/2
  w_max/1 -> Subtract1/1
  Constant/1 -> Subtract/2
  Subtract/1 -> Product1/1
  Divide/1 -> Math Function/1
  w_min/1 -> Add/2, Subtract1/2
  Product1/1 -> Product2/1  "K"
  Subtract1/1 -> Product2/2
  Product2/1 -> Add/1
  Sine Wave/1 -> Amplitude/1
  Add/1 -> Discrete-Time Integrator/1  "w"
  Discrete-Time Integrator/1 -> Sine Wave/1  "theta(t)"
  Amplitude/1 -> Sum/1
  Sum/1 -> chirp out/1
  Band-Limited White Noise/1 -> LPFilter/1
  Ground/1 -> Switch/3
  Switch/1 -> Sum/2  "white noise"
  LPFilter/1 -> Switch/1
  time/1 -> Saturation/1
  isNoiseOn/1 -> Switch/2

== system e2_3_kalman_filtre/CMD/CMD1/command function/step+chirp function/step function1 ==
  time : Inport
  Constant : Constant  Value=step_period+zero3_time
  Constant3 : Constant  Value=fcnCmdMag
  Constant4 : Constant  Value=0
  Gain : Gain  Gain=-1
  Saturation : Saturate  UpperLimit=inf  LowerLimit=0
  Subsystem : Subsystem
  Subsystem1 : Subsystem
  Subsystem2 : Subsystem
  Subsystem3 : Subsystem
  Subtract : Sum  Inputs=+-
  timeOut : Outport
  stepOut : Outport  Port=2
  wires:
  Saturation/1 -> timeOut/1
  Constant/1 -> Subtract/2
  Subtract/1 -> Saturation/1
  Subsystem3/1(timeOut) -> Subtract/1
  Subsystem2/2(Out) -> Subsystem3/2(0cmd)
  Subsystem2/1(timeOut) -> Subsystem3/1(time)
  Gain/1 -> Subsystem2/3(1cmd)
  Subsystem1/2(Out) -> Subsystem2/2(0cmd)
  Subsystem1/1(timeOut) -> Subsystem2/1(time)
  Subsystem/2(Out) -> Subsystem1/2(0cmd)
  Subsystem/1(timeOut) -> Subsystem1/1(time)
  Constant3/1 -> Gain/1, Subsystem/3(1cmd)
  Constant4/1 -> Subsystem/2(0cmd), Subsystem3/3(1cmd), Subsystem1/3(1cmd)
  Subsystem3/2(Out) -> stepOut/1
  time/1 -> Subsystem/1(time)

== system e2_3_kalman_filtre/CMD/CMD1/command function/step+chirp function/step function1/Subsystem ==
  time : Inport
  0cmd : Inport  Port=2
  1cmd : Inport  Port=3
  Divide : Product  Inputs=*/
  Switch : Switch  Threshold=1
  threshold : Constant  Value=zero1_time
  timeOut : Outport
  Out : Outport  Port=2
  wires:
  threshold/1 -> Divide/2
  Divide/1 -> Switch/2
  Switch/1 -> Out/1
  1cmd/1 -> Switch/1
  time/1 -> Divide/1, timeOut/1
  0cmd/1 -> Switch/3

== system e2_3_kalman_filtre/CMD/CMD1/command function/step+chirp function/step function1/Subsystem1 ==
  time : Inport
  0cmd : Inport  Port=2
  1cmd : Inport  Port=3
  Divide : Product  Inputs=*/
  Switch : Switch  Threshold=1
  threshold : Constant  Value=zero1_time+high_time
  timeOut : Outport
  Out : Outport  Port=2
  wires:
  0cmd/1 -> Switch/3
  time/1 -> timeOut/1, Divide/1
  1cmd/1 -> Switch/1
  Switch/1 -> Out/1
  Divide/1 -> Switch/2
  threshold/1 -> Divide/2

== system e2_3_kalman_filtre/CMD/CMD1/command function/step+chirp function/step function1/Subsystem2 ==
  time : Inport
  0cmd : Inport  Port=2
  1cmd : Inport  Port=3
  Divide : Product  Inputs=*/
  Switch : Switch  Threshold=1
  threshold : Constant  Value=zero1_time+high_time+zero2_time
  timeOut : Outport
  Out : Outport  Port=2
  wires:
  threshold/1 -> Divide/2
  Divide/1 -> Switch/2
  Switch/1 -> Out/1
  1cmd/1 -> Switch/1
  time/1 -> Divide/1, timeOut/1
  0cmd/1 -> Switch/3
